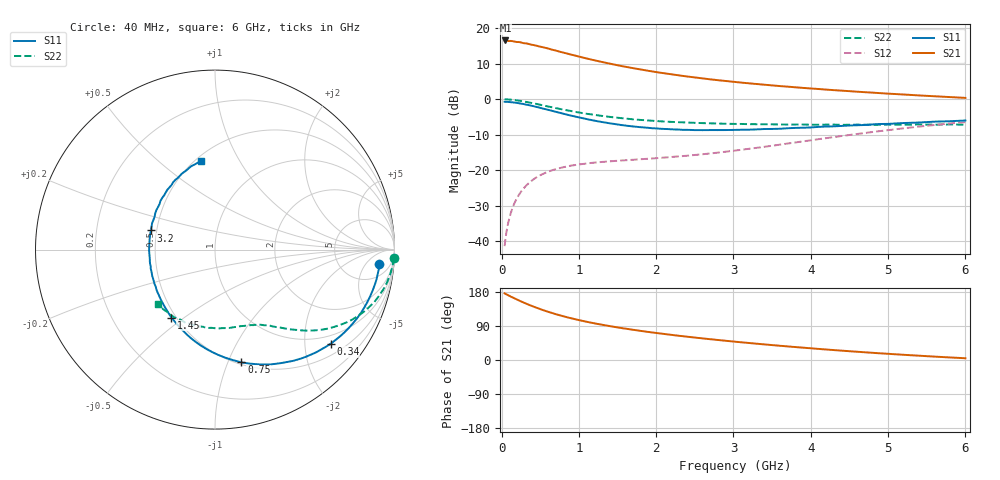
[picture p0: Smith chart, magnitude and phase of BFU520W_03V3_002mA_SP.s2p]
! Filename:  P:\Prog\Test\Noise\ATS_data\Testdata_Net\Run2\BFU520W_APM2013_06_A05_03p3V_002mA_SP_CM01_D.s2p
! Date/Time: Tue 26/Mar/2013 18:01:38
! BFU520W_APM2013_06_A05_03p3V_1to20mA_SP_CM01_Bias2_R.s2p
! MDIF S-parameter v. bias file
! BFU520W_APM2013_06_A05_03p3V_1to20mA_SP_CM01
! Date/time Tue Mar 19 16:47:37 2013
! VAR V_out= 3.3000
! VAR I_out= 2.0000
! VAR V_in= 0.8120
! VAR I_in= 0.0225
! Device data file deembeded for feedlines and parallel
! Original file: \Run2\BFU520W_APM2013_06_A05_03p3V_002mA_SP_CM01_R.s2p
! Feed-files: PR019V01_070313_Feed1.s2p, PR019V01_070313_Feed2.s2p
! Parallel-file: PR019V01_070313_Par.s2p
# MHz S MA R 50
!  Freq-MHz  S11-mag  S11-arg  S21-mag  S21-arg  S12-mag  S12-arg  S22-mag  S22-arg
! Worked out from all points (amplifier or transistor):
!   98 points, 40 MHz to 6 GHz, reference 50 ohm
!   highest |S21| = 16.5 dB at 50 MHz (marker M1)
!   |S21| within 3 dB of that: start of sweep to 726.3 MHz
!   unconditionally stable (mu >= 1): 2.337 GHz to 3.614 GHz
!   at 300 MHz: K = 0.18, MSG = 20.3 dB, |S12| = -24.8 dB
!   at 1.6 GHz: K = 0.79, MSG = 13.2 dB, |S12| = -17.2 dB
!   at 6 GHz: K = 0.83, MSG = 3.4 dB, |S12| = -6.4 dB
!   S11 on the Smith chart (normalised r, x): 40 MHz: 12, -12; 340 MHz: 0.77, -2.61; 750 MHz: 0.52, -1.12; 1.45 GHz: 0.47, -0.45; 3.2 GHz: 0.47, +0.12; 6 GHz: 0.53, +0.70
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40  0.9195 -4.8  6.704 175.8  0.00851 86.9  0.9964 -2.7
50  0.9195 -6.0  6.718 174.6  0.01056 86.2  0.997 -3.4
90  0.9144 -10.8  6.596 170.4  0.01881 83.2  0.9906 -6.3
120  0.9077 -14.4  6.62 167.4  0.02491 81.1  0.9848 -8.3
220  0.8788 -26.0  6.385 157.7  0.04398 74.4  0.9547 -14.8
340  0.831 -39.1  6.044 147.0  0.06385 67.2  0.9065 -21.7
420  0.7941 -47.3  5.777 140.4  0.07518 63.1  0.8713 -25.6
550  0.7315 -59.8  5.343 130.8  0.09006 57.4  0.8117 -31.2
600  0.7098 -64.5  5.19 127.4  0.095 55.6  0.7905 -33.0
750  0.6454 -76.8  4.674 118.2  0.1069 51.0  0.7312 -37.8
900  0.5871 -88.2  4.249 110.2  0.116 47.7  0.6813 -41.5
1050  0.5399 -98.5  3.863 103.1  0.1223 45.5  0.6361 -44.7
1250  0.4873 -111.1  3.436 94.9  0.1294 43.5  0.5916 -48.1
1450  0.4497 -122.7  3.087 87.7  0.1345 42.8  0.5554 -51.1
1750  0.4085 -138.3  2.679 78.4  0.1415 43.2  0.5158 -55.0
2050  0.3841 -152.5  2.363 70.1  0.149 44.8  0.489 -58.8
2500  0.3669 -171.8  2.025 59.2  0.1638 48.2  0.4648 -65.0
3100  0.3711 166.7  1.713 46.8  0.1937 53.1  0.4479 -74.2
3200  0.3721 163.3  1.673 44.9  0.2001 53.7  0.4452 -75.7
4100  0.4075 138.2  1.392 29.3  0.2735 55.6  0.4362 -92.6
5200  0.4616 113.7  1.164 13.8  0.389 49.7  0.4354 -116.4
6000  0.5012 98.9  1.043 4.6  0.4761 42.1  0.438 -136.0
